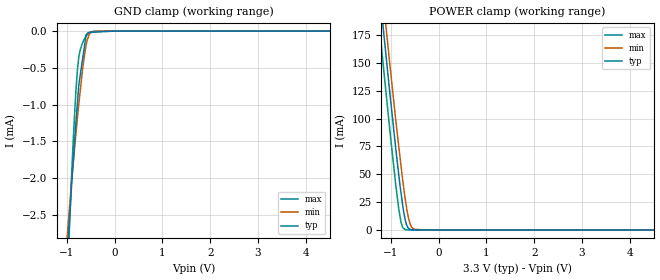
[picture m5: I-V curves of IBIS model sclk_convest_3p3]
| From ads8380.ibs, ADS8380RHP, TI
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|   sclk_convest_3p3 Model
[Model]   sclk_convest_3p3
Model_type   Input
Vinl = 0.8
Vinh = 2.3
|   typ   min   max
|   (nom PVT)   (fast PVT)   (slow PVT)
|C_comp from frequency sweep method (F=40MHz)
|Average
C_comp   9.728e-13   9.170e-13   9.808e-13
|C_comp from LC tank measurement(L=1nH)
|Average
|Resonant Frequency(Hz)   6.520e+09   6.870e+09   6.210e+09
|C_comp   5.965e-13   5.372e-13   6.575e-13
| Where nom  PVT is Nominal Process, 3.3V, 35C
|   Fast PVT is Strong Process,  3.6V, -40C
|   Slow PVT is Weak Process,   3V, 95C
[Model Spec]
Vinl   0.8   0.8   0.8
Vinh   2.3   2.0   2.6
[Voltage Range]   3.3   3   3.6
|Ambient Temperature   25   85   -40
|Junction Temperature
[Temperature Range]   35   95   -40
[Power Clamp Reference]   3.3   3   3.6
[GND Clamp Reference]   0   0   0
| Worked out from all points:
|   GND clamp passes 1 mA (typ) near -0.78 V on its own axis
|   POWER clamp passes 1 mA (typ) near -0.61 V on its own axis
[GND Clamp]
|   Voltage   I(typ)   I(min)   I(max)
-3.3V     -29.5mA    -22.08mA   -346.9mA
-1.48V    -8.435mA   -6.749mA   -11.2mA
-897.6mV  -2.079mA   -2.033mA   -1.938mA
-813.6mV  -1.291mA   -1.432mA   -869.3uA
-781.2mV  -1.016mA   -1.213mA   -563uA
-752.4mV  -772.5uA   -1.02mA    -377.4uA
-666mV    -368uA     -504.3uA   -154.1uA
-594mV    -49.28uA   -188.5uA   -63.98uA
-547.8mV  -18.81uA   -78.25uA   -34.03uA
-483mV    -16.57uA   -13.84uA   -10.13uA
-285mV    -9.73uA    -61.45nA   -1.03uA
6.6V      0A         0A         0A
[POWER Clamp]
|   Voltage   I(typ)   I(min)   I(max)
-3.3V     1.135A     1.155A     1.11A
-1.318V   249.1mA    274.8mA    216.8mA
-1.176V   187.9mA    213.6mA    155.3mA
-1.13V    168.7mA    194.3mA    135.5mA
-1.023V   123.4mA    149.3mA    90.46mA
-896.4mV  72.45mA    98.1mA     40mA
-835.2mV  49.7mA     75.13mA    19.03mA
-784.8mV  32.38mA    56.22mA    6.372mA
-691.2mV  7.748mA    25.44mA    159.7uA
-597mV    508.4uA    5.363mA    2.122uA
-516mV    127uA      660uA      747.1nA
6.6V      0A         0A         0A
